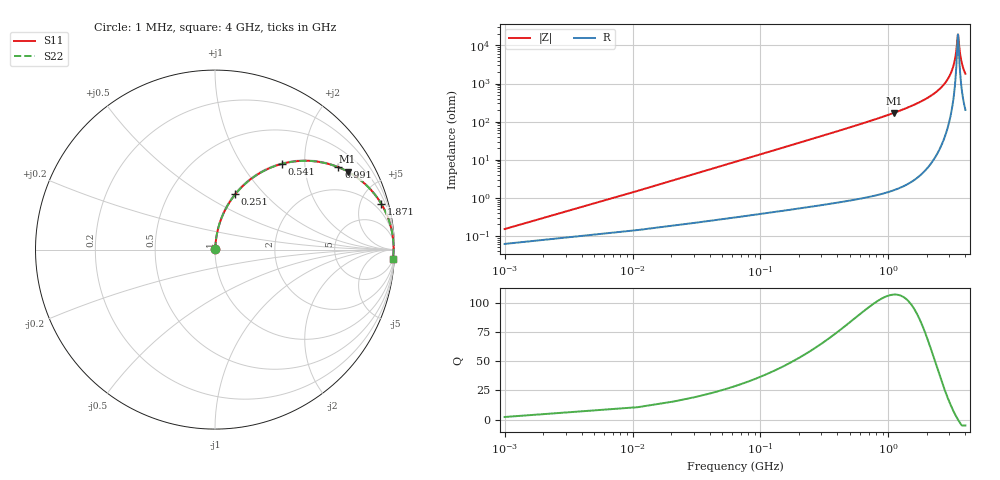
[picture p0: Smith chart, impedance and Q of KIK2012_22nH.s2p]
!version-2
!date-01.2022
!Series
# MHz S RI R 50
!Freq ReS11 ImS11 ReS21 ImS21 ReS12 ImS12 ReS22 ImS22
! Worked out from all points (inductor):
!   401 points, 1 MHz to 4 GHz, reference 50 ohm
!   read as one part in series: L = 22 nH near 21 MHz
!   highest Q = 107 at 1.101 GHz (marker M1), where L = 24.4 nH
!   self-resonance near 3.491 GHz
!   S11 on the Smith chart (normalised r, x): 1 MHz: 1.00, +0.00; 251 MHz: 1.01, +0.70; 541 MHz: 1.02, +1.53; 991 MHz: 1.03, +2.98; 1.871 GHz: 1.09, +7.24; 4 GHz: 5, -36
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1  0.000618 0.00138  0.9994 -0.00138  0.9994 -0.00138  0.000618 0.00138
31  0.00403 0.0426  0.996 -0.0426  0.996 -0.0426  0.00403 0.0426
61  0.00999 0.0833  0.99 -0.0833  0.99 -0.0833  0.00999 0.0833
131  0.0357 0.1741  0.9643 -0.1741  0.9643 -0.1741  0.0357 0.1741
251  0.1125 0.3077  0.8875 -0.3077  0.8875 -0.3077  0.1125 0.3077
541  0.3713 0.4774  0.6287 -0.4774  0.6287 -0.4774  0.3713 0.4774
671  0.4813 0.4944  0.5187 -0.4944  0.5187 -0.4944  0.4813 0.4944
991  0.6876 0.4588  0.3124 -0.4588  0.3124 -0.4588  0.6876 0.4588
1101  0.7385 0.4348  0.2615 -0.4348  0.2615 -0.4348  0.7385 0.4348
1341  0.8228 0.377  0.1772 -0.377  0.1772 -0.377  0.8228 0.377
1871  0.9264 0.2549  0.0736 -0.2549  0.0736 -0.2549  0.9264 0.2549
2001  0.9412 0.2283  0.0588 -0.2283  0.0588 -0.2283  0.9412 0.2283
2671  0.9837 0.1109  0.0163 -0.1109  0.0163 -0.1109  0.9837 0.1109
3091  0.993 0.051  0.00699 -0.051  0.00699 -0.051  0.993 0.051
3231  0.9943 0.0328  0.0057 -0.0328  0.0057 -0.0328  0.9943 0.0328
3341  0.9948 0.0191  0.00518 -0.0191  0.00518 -0.0191  0.9948 0.0191
3481  0.9949 0.00229  0.0051 -0.00229  0.0051 -0.00229  0.9949 0.00229
3501  0.9949 -5.5e-05  0.00513 5.5e-05  0.00513 5.5e-05  0.9949 -5.5e-05
3621  0.9944 -0.0138  0.00558 0.0138  0.00558 0.0138  0.9944 -0.0138
3701  0.9939 -0.0228  0.00608 0.0228  0.00608 0.0228  0.9939 -0.0228
3831  0.9928 -0.0368  0.00722 0.0368  0.00722 0.0368  0.9928 -0.0368
4000  0.9907 -0.0544  0.00925 0.0544  0.00925 0.0544  0.9907 -0.0544
